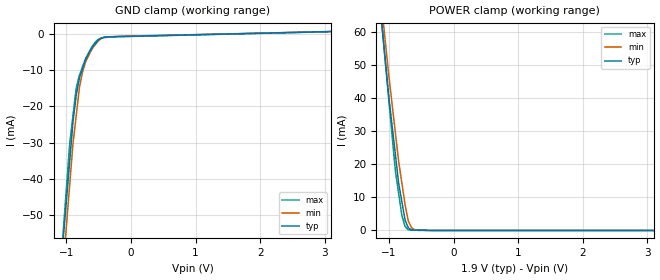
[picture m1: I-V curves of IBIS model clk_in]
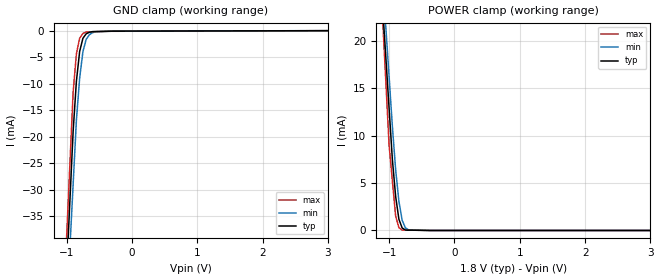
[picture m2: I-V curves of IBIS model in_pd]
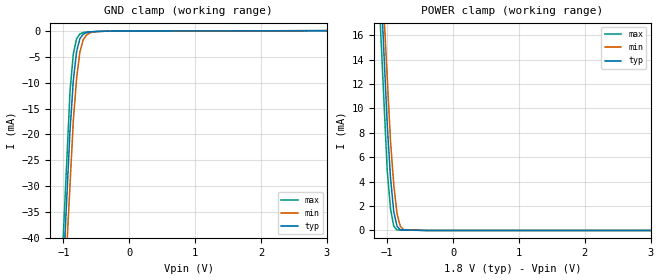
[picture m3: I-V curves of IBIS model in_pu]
| Teraspeed Modeling Services.
| http://www.teraspeedlabs.com
[IBIS Ver] 4.0
[File Name] ads58j89rgc.ibs
[File Rev] 3.0
[Date]   03-20-2015
[Notes]  Quality Check of this IBIS model: Model Passes IBIS Check. Model
   parses into ICX IS. Simulates with Hyperlynx.
   1. MIN TYP MAX information is based on Temperature and Voltage
   characteristics only.
   2. Package information extracted using Tektronix IConnect Software.
[Disclaimer]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
[Source]
| This model file was created by Teraspeed Labs LLC
| (http://www.teraspeedlabs.com/).
[Disclaimer]
| This product is designed as an aid for customers of Texas Instruments.
| No warranties, either expressed or implied, with respect to this third
| party software (if any) or with respect to its fitness for any
| particular purpose is claimed by Texas Instruments or the author. The
| software (if any) is provided solely on an "as is" basis. The entire
| risk as to its quality and performance is with the customer
[Copyright]
| (C) Copyright 2015 Texas Instruments Incorporated. All rights reserved.
| All other rights are reserved.
[Component] DAC58J89RGC
[Manufacturer] TI
| Data Sheet: SBAS659--NOVEMBER 2014
[Package]
| RGC(S-PVQFN-N64)/64 Lead QFN
| variable   typ   min   max
R_pkg  1.766E-02   1.490E-02   2.060E-02
L_pkg  1.591E-09   1.340E-09   1.850E-09
C_pkg  4.418E-13   3.720E-13   5.150E-13
[Pin] signal_name  model_name  R_pin  L_pin C_pin
1   SDOUT   spi_tri   2.060E-02   1.850E-09   5.150E-13
2   SDATA   spi_io   1.970E-02   1.780E-09   4.930E-13
3   SCLK   in_pd   1.890E-02   1.700E-09   4.720E-13
4   SDENb   in_pd   1.800E-02   1.620E-09   4.510E-13
5   SYSREFABM   sysref   1.720E-02   1.550E-09   4.300E-13
6   SYSREFABP   sysref   1.640E-02   1.480E-09   4.100E-13
7   AVDDC   POWER   1.560E-02   1.410E-09   3.910E-13
8   CLKINM   clk_in   1.490E-02   1.340E-09   3.720E-13
9   CLKINP   clk_in   1.490E-02   1.340E-09   3.720E-13
10   AVDDC   POWER   1.560E-02   1.410E-09   3.910E-13
11   SYSREFCDP   sysref   1.640E-02   1.480E-09   4.100E-13
12   SYSREFCDM   sysref   1.720E-02   1.550E-09   4.300E-13
13   SRESETb   in_pu   1.800E-02   1.620E-09   4.510E-13
14   ENABLE   in_pd   1.890E-02   1.700E-09   4.720E-13
15   VREF   term   1.970E-02   1.780E-09   4.930E-13
16   VCM   term   2.060E-02   1.850E-09   5.150E-13
17   AVDD33   POWER   2.060E-02   1.850E-09   5.150E-13
18   INCP   adc_in   1.970E-02   1.780E-09   4.930E-13
19   INCM   adc_in   1.890E-02   1.700E-09   4.720E-13
20   AVDD33   POWER   1.800E-02   1.620E-09   4.510E-13
21   AVDD18   POWER   1.720E-02   1.550E-09   4.300E-13
22   INDM   adc_in   1.640E-02   1.480E-09   4.100E-13
23   INDP   adc_in   1.560E-02   1.410E-09   3.910E-13
24   AVDD18   POWER   1.490E-02   1.340E-09   3.720E-13
25   DVDD   POWER   1.490E-02   1.340E-09   3.720E-13
26   DC0P   term   1.560E-02   1.410E-09   3.910E-13
27   DC0M   term   1.640E-02   1.480E-09   4.100E-13
28   IOVDD   POWER   1.720E-02   1.550E-09   4.300E-13
29   DC1P   term   1.800E-02   1.620E-09   4.510E-13
30   DC1M   term   1.890E-02   1.700E-09   4.720E-13
31   OVRC   ovr_io   1.970E-02   1.780E-09   4.930E-13
32   OVRD   ovr_tri   2.060E-02   1.850E-09   5.150E-13
33   SYNCbCDM   lvds_in   2.060E-02   1.850E-09   5.150E-13
34   SYNCbCDP   lvds_in   1.970E-02   1.780E-09   4.930E-13
35   DD0P   term   1.890E-02   1.700E-09   4.720E-13
36   DD0M   term   1.800E-02   1.620E-09   4.510E-13
37   IOVDD   POWER   1.720E-02   1.550E-09   4.300E-13
38   DD1P   term   1.640E-02   1.480E-09   4.100E-13
39   DD1M   term   1.560E-02   1.410E-09   3.910E-13
40   PLLVDD   POWER   1.490E-02   1.340E-09   3.720E-13
41   PLLVDD   POWER   1.490E-02   1.340E-09   3.720E-13
42   DB1M   term   1.560E-02   1.410E-09   3.910E-13
43   DB1P   term   1.640E-02   1.480E-09   4.100E-13
44   IOVDD   POWER   1.720E-02   1.550E-09   4.300E-13
45   DB0M   term   1.800E-02   1.620E-09   4.510E-13
46   DB0P   term   1.890E-02   1.700E-09   4.720E-13
47   SYNCbABP   lvds_in   1.970E-02   1.780E-09   4.930E-13
48   SYNCbABM   lvds_in   2.060E-02   1.850E-09   5.150E-13
49   OVRB   ovr_tri   2.060E-02   1.850E-09   5.150E-13
50   OVRA   ovr_io   1.970E-02   1.780E-09   4.930E-13
51   DA1M   term   1.890E-02   1.700E-09   4.720E-13
52   DA1P   term   1.800E-02   1.620E-09   4.510E-13
53   IOVDD   POWER   1.720E-02   1.550E-09   4.300E-13
54   DA0M   term   1.640E-02   1.480E-09   4.100E-13
55   DA0P   term   1.560E-02   1.410E-09   3.910E-13
56   DVDD   POWER   1.490E-02   1.340E-09   3.720E-13
57   AVDD18   POWER   1.490E-02   1.340E-09   3.720E-13
58   INBP   adc_in   1.560E-02   1.410E-09   3.910E-13
59   INBM   adc_in   1.640E-02   1.480E-09   4.100E-13
60   AVDD18   POWER   1.720E-02   1.550E-09   4.300E-13
61   AVDD33   POWER   1.800E-02   1.620E-09   4.510E-13
62   INAM   adc_in   1.890E-02   1.700E-09   4.720E-13
63   INAP   adc_in   1.970E-02   1.780E-09   4.930E-13
64   AVDD33   POWER   2.060E-02   1.850E-09   5.150E-13
65   GND_PAD   GND   0.000E+00   0.000E+00   0.000E+00
[Diff Pin] inv_pin vdiff tdelay_typ tdelay_min  tdelay_max
9   8   400mV   NA   NA   NA
47   48   350mV   NA   NA   NA
34   33   350mV   NA   NA   NA
| Pairs to be selectively commented out when sysref in SE mode
6   5   350mV   NA   NA   NA
11   12   350mV   NA   NA   NA
[Series Pin Mapping]   pin_2   model_name
6   5   100ohm
11   12   100ohm
34   33   100ohm
47   48   100ohm
[Model Selector] sysref
lvds_in   lvds sysref input,differential
sysref_se   sysref input,single ended
[Model]  100ohm
Model_type Series
C_comp   0   0   0
[Voltage Range]  1.80   1.70   1.90
[Temperature Range]   25   85   -40
[R series]   100   80   120
[Model]  term
Model_type Terminator
C_comp   0   0   0
[Voltage Range]  1.90  1.80  2.00
[Temperature Range]   25   85   -40
| Models and submodels in the file (12): clk_in (Input), in_pd (Input), in_pu (Input), lvds_in (Input), sysref_se (Input), ovr_io (I/O), ovr_tri (3-state), spi_io (I/O), spi_tri (3-state), 100ohm (Series), adc_in (Terminator), term (Terminator)
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[Model] clk_in
Model_type Input
Vinl = 700.000mV
Vinh = 1.10000V
C_comp 1.11000pF 1.09000pF 1.13000pF
| variable typ   min   max
[Voltage Range] 1.90000V 1.80000V 2.00000V
[POWER Clamp Reference] 1.90000V 1.80000V 2.00000V
[GND Clamp Reference] 0.00000V 0.00000V 0.00000V
[Temperature Range]   25   85   -40
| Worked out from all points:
|   GND clamp passes 1 mA (typ) near -0.41 V on its own axis
|   POWER clamp passes 1 mA (typ) near -0.70 V on its own axis
[GND Clamp]
-1.9V     -238.2mA   -254mA     -260.7mA
-950mV    -35.19mA   -41.7mA    -30.37mA
-900mV    -24.51mA   -30.53mA   -22.74mA
-850mV    -17.13mA   -22.76mA   -15.11mA
-800mV    -12.32mA   -14.99mA   -11.48mA
-750mV    -9.638mA   -10.5mA    -9.103mA
-700mV    -6.954mA   -7.63mA    -6.728mA
-600mV    -3.732mA   -4.103mA   -3.481mA
-500mV    -1.66mA    -1.875mA   -1.506mA
-400mV    -950.9uA   -957.8uA   -1.063mA
-200mV    -813.1uA   -771.3uA   -862uA
3.8V      848.7uA    859.3uA    824.5uA
[POWER Clamp]
-1.9V     223.9mA    215.2mA    227.9mA
-1V       39.96mA    46.4mA     38.94mA
-900mV    22.88mA    29.37mA    17.95mA
-850mV    14.33mA    20.86mA    11.24mA
-800mV    8.718mA    14.32mA    4.53mA
-750mV    3.101mA    7.785mA    1.203mA
-700mV    826.5uA    2.793mA    183uA
-650mV    133uA      817.7uA    160.1uA
-600mV    112.5uA    209.2uA    137.3uA
-550mV    92.08uA    33.73uA    114.4uA
3.8V      0A         0A         0A
[Model] in_pd
Model_type Input
Vinl = 400.000mV
Vinh = 1.20000V
C_comp 663.000fF 661.000fF 665.000fF
| variable typ   min   max
[Voltage Range] 1.80000V 1.70000V 1.90000V
[POWER Clamp Reference] 1.80000V 1.70000V 1.90000V
[GND Clamp Reference] 0.00000V 0.00000V 0.00000V
[Temperature Range]   25   85   -40
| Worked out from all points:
|   GND clamp passes 1 mA (typ) near -0.73 V on its own axis
|   POWER clamp passes 1 mA (typ) near -0.84 V on its own axis
[GND Clamp]
-1.8V     -257.5mA   -247mA     -258.3mA
-900mV    -18.96mA   -28.98mA   -11.57mA
-850mV    -9.489mA   -16.86mA   -4.313mA
-800mV    -3.845mA   -8.862mA   -1.361mA
-750mV    -1.371mA   -3.886mA   -461.4uA
-700mV    -521uA     -1.562mA   -191.7uA
-650mV    -239.7uA   -696.9uA   -171.5uA
-600mV    -111.2uA   -302.8uA   -151.4uA
-550mV    -97.03uA   -139uA     -131.3uA
3.6V      77.72uA    83.77uA    82.51uA
[POWER Clamp]
-1.8V     113.7mA    103.8mA    116.7mA
-1.1V     23.63mA    26.61mA    22.43mA
-1V       12.87mA    16.2mA     8.964mA
-950mV    7.488mA    11mA       5.245mA
-900mV    3.603mA    6.41mA     1.527mA
-850mV    1.184mA    3.074mA    303uA
-800mV    262.2uA    1.075mA    44.66uA
-750mV    43.19uA    268.6uA    39.7uA
-700mV    37.43uA    63.8uA     34.74uA
3.6V      0A         0A         0A
[Model] in_pu
Model_type Input
Vinl = 400.000mV
Vinh = 1.20000V
C_comp 548.000fF 526.000fF 570.000fF
| variable typ   min   max
[Voltage Range] 1.80000V 1.70000V 1.90000V
[POWER Clamp Reference] 1.80000V 1.70000V 1.90000V
[GND Clamp Reference] 0.00000V 0.00000V 0.00000V
[Temperature Range]   25   85   -40
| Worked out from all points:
|   GND clamp passes 1 mA (typ) near -0.72 V on its own axis
|   POWER clamp passes 1 mA (typ) near -0.88 V on its own axis
[GND Clamp]
-1.8V     -259.5mA   -251.4mA   -257.7mA
-900mV    -19.16mA   -29.65mA   -11.62mA
-850mV    -9.611mA   -17.33mA   -4.423mA
-800mV    -3.976mA   -9.133mA   -1.511mA
-750mV    -1.509mA   -4.08mA    -610.6uA
-700mV    -650.3uA   -1.713mA   -328.9uA
-650mV    -356.4uA   -822.7uA   -225.5uA
-600mV    -215.9uA   -409.6uA   -200.8uA
-450mV    -96.77uA   -101.2uA   -126.6uA
3.6V      38.03uA    44.13uA    46.58uA
[POWER Clamp]
-1.8V     102.6mA    96.49mA    115.8mA
-1.1V     20.47mA    23.08mA    16.41mA
-1.05V    14.6mA     17.84mA    10.68mA
-1V       8.732mA    12.6mA     4.951mA
-950mV    4.339mA    7.353mA    1.789mA
-900mV    1.522mA    3.714mA    347.8uA
-850mV    331.7uA    1.344mA    39.23uA
-800mV    53.76uA    333.3uA    35.1uA
-750mV    47.04uA    63.82uA    30.97uA
-400mV    0A         0A         2.065uA
3.6V      0A         0A         0A
